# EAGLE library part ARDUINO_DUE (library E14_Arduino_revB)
Device for representing an Arduino Due board with a footprint in an EAGLE design. Created by Dave Young for Element14. More EAGLE documentation at: http://www.element14.com/community/community/knode/cadsoft_eagle
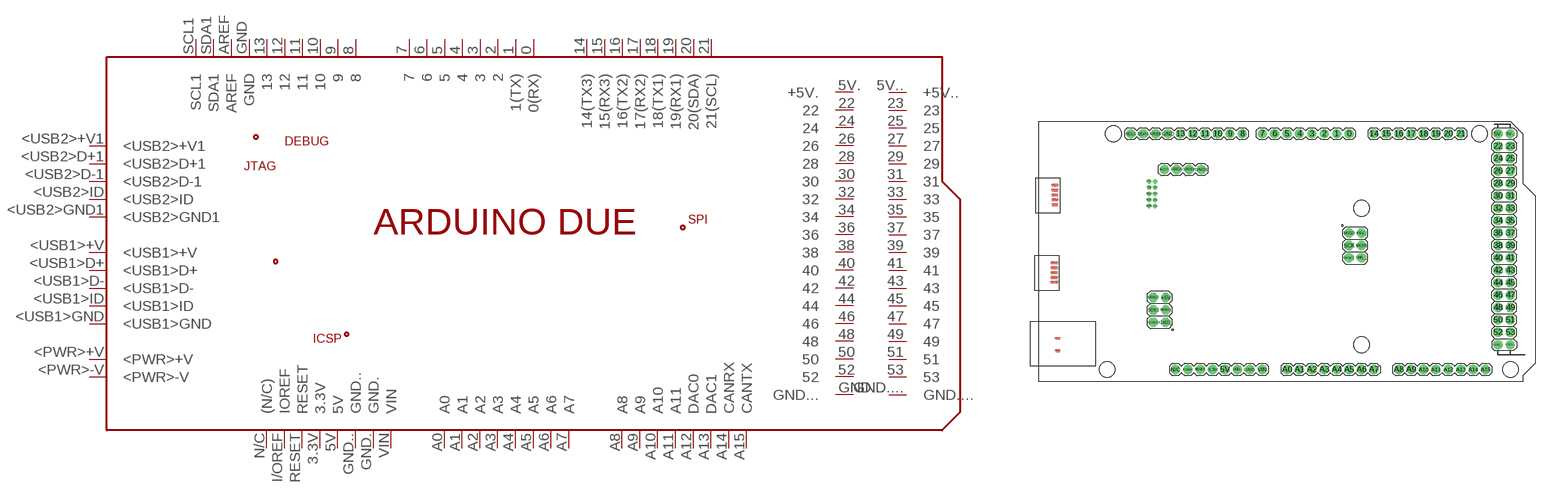
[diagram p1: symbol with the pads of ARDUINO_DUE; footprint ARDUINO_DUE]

Designator prefix PCB

## ARDUINO_DUE  [ARDUINO_DUE]
0  0(RX)
1  1(TX)
2  2
3  3
3.3V  3.3V
4  4
5  5
5V  5V
5V.  +5V.
5V..  +5V..
6  6
7  7
8  8
9  9
10  10
11  11
12  12
13  13
14  14(TX3)
15  15(RX3)
16  16(TX2)
17  17(RX2)
18  18(TX1)
19  19(RX1)
20  20(SDA)
21  21(SCL)
22  22
23  23
24  24
25  25
26  26
27  27
28  28
29  29
30  30
31  31
32  32
33  33
34  34
35  35
36  36
37  37
38  38
39  39
40  40
41  41
42  42
43  43
44  44
45  45
46  46
47  47
48  48
49  49
50  50
51  51
52  52
53  53
+3.3V  +3.3V
+5V  +5V
+5V_  +5V_
<PWR>+V  <PWR>+V
<PWR>-V  <PWR>-V
<USB1>+V  <USB1>+V
<USB1>D+  <USB1>D+
<USB1>D-  <USB1>D-
<USB1>GND  <USB1>GND
<USB1>ID  <USB1>ID
<USB2>+V1  <USB2>+V1
<USB2>D+1  <USB2>D+1
<USB2>D-1  <USB2>D-1
<USB2>GND1  <USB2>GND1
<USB2>ID  <USB2>ID
A0  A0
A1  A1
A2  A2
A3  A3
A4  A4
A5  A5
A6  A6
A7  A7
A8  A8
A9  A9
A10  A10
A11  A11
A12  DAC0
A13  DAC1
A14  CANRX
A15  CANTX
AREF  AREF
GND  GND
GND1  GND1
GND1.  GND1.
GND1..  GND1..
GND1...  GND1...
GND.  GND.
GND..  GND..
GND...  GND...
GND....  GND....
GND_  GND_
GND__  GND__
I/OREF  IOREF
MISO  MISO
MISO2  MISO2
MOSI  MOSI
MOSI2  MOSI2
N/C  (N/C)
N/C.  N/C.
RESET  RESET
RESET2  RESET2
RESET.  RESET.
RESET..  RESET..
RESET_  RESET_
SCK  SCK
SCK2  SCK2
SCL1  SCL1
SDA1  SDA1
SWCLK  SWCLK
SWDIO  SWDIO
TCK  TCK
TDI  TDI
TDO  TDO
TMS  TMS
VIN  VIN

## Footprint ARDUINO_DUE (pad centres in mm)
Footprint for representing an Arduino Due board in an EAGLE schematic. Created by Dave Young for Element14. More EAGLE documentation at: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
drill 1.016 pad 1.88: 0 63.5,50.8; 1 60.96,50.8; 2 58.42,50.8; 3 55.88,50.8; 3.3V 35.56,2.54; 4 53.34,50.8; 5 50.8,50.8; 5V 38.1,2.54; 5V. 93.98,50.8; 5V.. 96.52,50.8; 6 48.26,50.8; 7 45.72,50.8; 8 41.656,50.8; 9 39.116,50.8; 10 36.576,50.8; 11 34.036,50.8; 12 31.496,50.8; 13 28.956,50.8; 14 68.58,50.8; 15 71.12,50.8; 16 73.66,50.8; 17 76.2,50.8; 18 78.74,50.8; 19 81.28,50.8; 20 83.82,50.8; 21 86.36,50.8; A0 50.8,2.54; A1 53.34,2.54; A2 55.88,2.54; A3 58.42,2.54; A4 60.96,2.54; A5 63.5,2.54; A6 66.04,2.54; A7 68.58,2.54; A8 73.66,2.54; A9 76.2,2.54; A10 78.74,2.54; A11 81.28,2.54; A12 83.82,2.54; A13 86.36,2.54; A14 88.9,2.54; A15 91.44,2.54; AREF 23.876,50.8; GND 26.416,50.8; GND1 33.274,43.485; GND. 43.18,2.54; GND.. 40.64,2.54; GND... 93.98,7.62; GND.... 96.52,7.62; I/OREF 30.48,2.54; N/C 27.94,2.54; RESET 33.02,2.54; RESET.. 25.654,43.485; SCL1 18.796,50.8; SDA1 21.336,50.8; SWCLK 30.734,43.485; SWDIO 28.194,43.485; VIN 45.72,2.54
drill 1.016 pad 1.88 octagon: 22 93.98,48.26; 23 96.52,48.26; 24 93.98,45.72; 25 96.52,45.72; 26 93.98,43.18; 27 96.52,43.18; 28 93.98,40.64; 29 96.52,40.64; 30 93.98,38.1; 31 96.52,38.1; 32 93.98,35.56; 33 96.52,35.56; 34 93.98,33.02; 35 96.52,33.02; 36 93.98,30.48; 37 96.52,30.48; 38 93.98,27.94; 39 96.52,27.94; 40 93.98,25.4; 41 96.52,25.4; 42 93.98,22.86; 43 96.52,22.86; 44 93.98,20.32; 45 96.52,20.32; 46 93.98,17.78; 47 96.52,17.78; 48 93.98,15.24; 49 96.52,15.24; 50 93.98,12.7; 51 96.52,12.7; 52 93.98,10.16; 53 96.52,10.16; +5V 25.959,17.272; +5V_ 66.04,30.48; GND_ 25.959,12.192; GND__ 66.04,25.4; MISO 63.5,30.48; MISO2 23.419,17.272; MOSI 66.04,27.94; MOSI2 25.959,14.732; RESET2 23.419,12.192; RESET. 63.5,25.4; SCK 63.5,27.94; SCK2 23.419,14.732
drill 0.406 pad 0.61: +3.3V 23.8,35.966; GND1. 23.8,37.236; GND1.. 23.8,38.506; GND1... 23.8,41.046; N/C. 23.8,39.776; RESET_ 22.53,41.046; TCK 22.53,37.236; TDI 22.53,39.776; TDO 22.53,38.506; TMS 22.53,35.966
smd 1.016 x 0.508: <PWR>+V 3.81,8.89; <PWR>-V 3.81,6.35
smd 1.27 x 0.635: <USB1>+V 3.099,24.359; <USB1>D+ 3.099,23.368; <USB1>D- 3.099,22.352; <USB1>GND 3.099,20.371; <USB1>ID 3.099,21.387; <USB2>+V1 3.302,40.234; <USB2>D+1 3.302,39.243; <USB2>D-1 3.302,38.227; <USB2>GND1 3.302,36.246; <USB2>ID 3.302,37.262
hole 3.2 at 15.24,50.8
hole 3.2 at 13.97,2.54
hole 3.2 at 66.04,35.56
hole 3.2 at 66.04,7.62
hole 3.2 at 90.17,50.8
hole 3.2 at 96.52,2.54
